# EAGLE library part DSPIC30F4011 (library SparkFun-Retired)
Microchip 16-bit DSP for UAVv2x SparkFun Products None Not tested
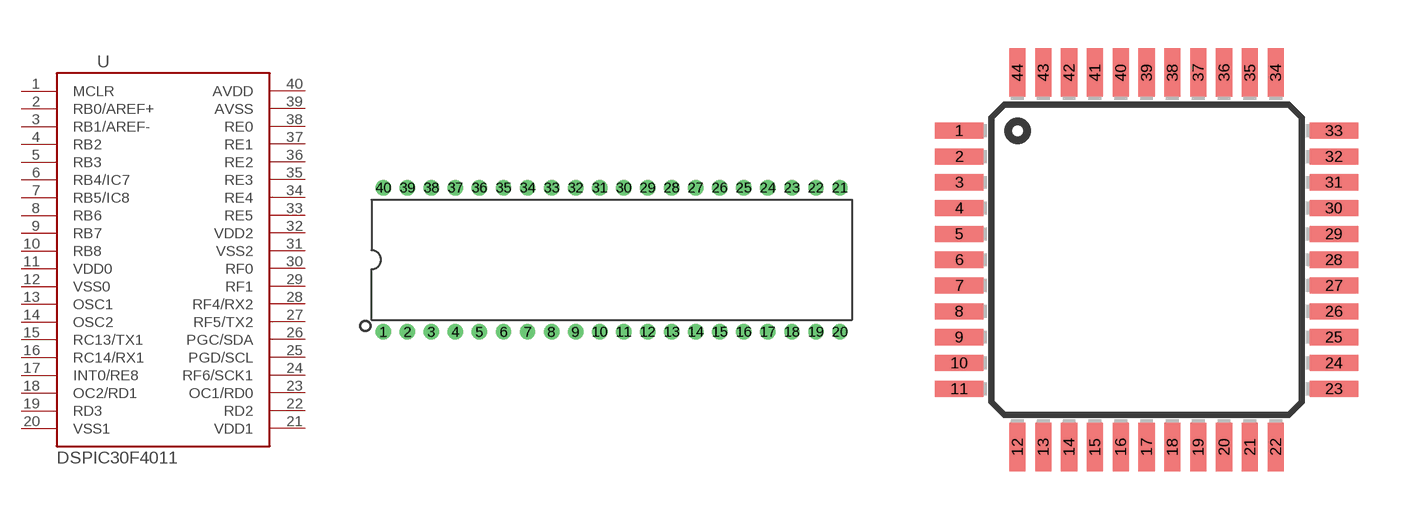
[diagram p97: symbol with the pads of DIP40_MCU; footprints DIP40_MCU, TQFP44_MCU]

Designator prefix -

## DSPIC30F4011DIL  [DIP40_MCU]
1  MCLR
2  RB0/AREF+
3  RB1/AREF-
4  RB2
5  RB3
6  RB4/IC7
7  RB5/IC8
8  RB6
9  RB7
10  RB8
11  VDD0
12  VSS0
13  OSC1
14  OSC2
15  RC13/TX1
16  RC14/RX1
17  INT0/RE8
18  OC2/RD1
19  RD3
20  VSS1
21  VDD1
22  RD2
23  OC1/RD0
24  RF6/SCK1
25  PGD/SCL
26  PGC/SDA
27  RF5/TX2
28  RF4/RX2
29  RF1
30  RF0
31  VSS2
32  VDD2
33  RE5
34  RE4
35  RE3
36  RE2
37  RE1
38  RE0
39  AVSS
40  AVDD

## DSPIC30F4011  [TQFP44_MCU]
1  PGC/SDA
2  RF5/TX2
3  RF4/RX2
4  RF1
5  RF0
6  VSS0
7  VDD0
8  RE5
9  RE4
10  RE3
11  RE2
14  RE1
15  RE0
16  AVSS
17  AVDD
18  MCLR
19  RB0/AREF+
20  RB1/AREF-
21  RB2
22  RB3
23  RB4/IC7
24  RB5/IC8
25  RB6
26  RB7
27  RB8
28  VDD1
29  VSS1
30  OSC1
31  OSC2
32  RC13/TX1
35  RC14/RX1
36  INT0/RE8
37  OC2/RD1
38  RD3
39  VSS2
40  VDD2
41  RD2
42  OC1/RD0
43  RF6/SCK1
44  PGD/SCL

## Footprint DIP40_MCU (pad centres in mm)
Dual In Line Package: 40-pin PDIP
drill 0.813 pad 1.626: 1 -24.13,-7.62; 2 -21.59,-7.62; 3 -19.05,-7.62; 4 -16.51,-7.62; 5 -13.97,-7.62; 6 -11.43,-7.62; 7 -8.89,-7.62; 8 -6.35,-7.62; 9 -3.81,-7.62; 10 -1.27,-7.62; 11 1.27,-7.62; 12 3.81,-7.62; 13 6.35,-7.62; 14 8.89,-7.62; 15 11.43,-7.62; 16 13.97,-7.62; 17 16.51,-7.62; 18 19.05,-7.62; 19 21.59,-7.62; 20 24.13,-7.62; 21 24.13,7.62; 22 21.59,7.62; 23 19.05,7.62; 24 16.51,7.62; 25 13.97,7.62; 26 11.43,7.62; 27 8.89,7.62; 28 6.35,7.62; 29 3.81,7.62; 30 1.27,7.62; 31 -1.27,7.62; 32 -3.81,7.62; 33 -6.35,7.62; 34 -8.89,7.62; 35 -11.43,7.62; 36 -13.97,7.62; 37 -16.51,7.62; 38 -19.05,7.62; 39 -21.59,7.62; 40 -24.13,7.62

## Footprint TQFP44_MCU (pad centres in mm)
smd 1.5 x 0.5: 1 -5.8,4; 2 -5.8,3.2; 3 -5.8,2.4; 4 -5.8,1.6; 5 -5.8,0.8; 6 -5.8,0; 7 -5.8,-0.8; 8 -5.8,-1.6; 9 -5.8,-2.4; 10 -5.8,-3.2; 11 -5.8,-4; 23 5.8,-4; 24 5.8,-3.2; 25 5.8,-2.4; 26 5.8,-1.6; 27 5.8,-0.8; 28 5.8,0; 29 5.8,0.8; 30 5.8,1.6; 31 5.8,2.4; 32 5.8,3.2; 33 5.8,4
smd 0.5 x 1.5: 12 -4,-5.8; 13 -3.2,-5.8; 14 -2.4,-5.8; 15 -1.6,-5.8; 16 -0.8,-5.8; 17 0,-5.8; 18 0.8,-5.8; 19 1.6,-5.8; 20 2.4,-5.8; 21 3.2,-5.8; 22 4,-5.8; 34 4,5.8; 35 3.2,5.8; 36 2.4,5.8; 37 1.6,5.8; 38 0.8,5.8; 39 0,5.8; 40 -0.8,5.8; 41 -1.6,5.8; 42 -2.4,5.8; 43 -3.2,5.8; 44 -4,5.8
